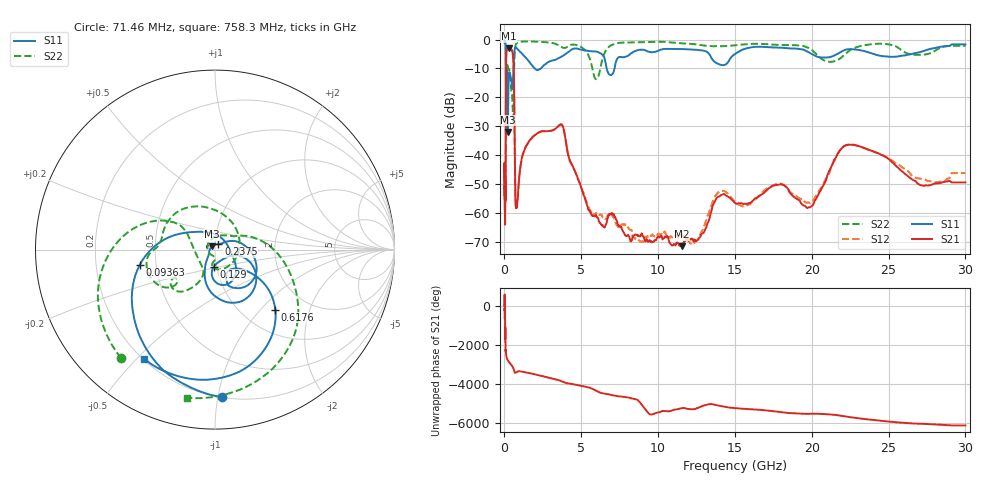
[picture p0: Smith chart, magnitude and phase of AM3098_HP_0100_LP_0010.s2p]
! Date/Time: Thu, Feb 28, 2019 8:35 AM
! Network Analyzer: Agilent Technologies E8364B Rev: A.07.50.67
! Sweep from 0.010 to 30.000 GHz, 1601 Points, Sweep Type: LOG
! Power Supply: 5.022 V, 0.002 A
# Hz S DB R 50
!freq MagS11 AngS11 MagS21 AngS21 MagS12 AngS12 MagS22 AngS22
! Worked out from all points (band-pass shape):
!   1601 points, 10 MHz to 30 GHz, reference 50 ohm
!   highest |S21| = -3.03 dB at 269.1 MHz (marker M1); lowest = -71.5 dB at 11.54 GHz (marker M2)
!   |S21| within 3 dB of the highest: 111.2 MHz to 562.7 MHz (451.5 MHz wide, 134 % of centre)
!   lowest |S11| = -32.0 dB at 229.3 MHz (marker M3), VSWR 1.05, Z = 48.3 + j1.78 ohm
!   |S11| at or under -10 dB: 176.3 MHz to 588 MHz (411.7 MHz wide, 108 % of centre); 1.966 GHz to 2.381 GHz (415.1 MHz wide, 19.1 % of centre); 6.65 GHz to 7.164 GHz (513.4 MHz wide, 7.43 % of centre)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
!   |S22| runs from -28.9 to -0.5 dB; largest |S21 - S12| = 0.012
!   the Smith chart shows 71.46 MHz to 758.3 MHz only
!   S11 on the Smith chart (normalised r, x): 71.46 MHz: 0.20, -1.03; 93.63 MHz: 0.40, -0.09; 129 MHz: 0.97, -0.19; 237.5 MHz: 1.04, +0.06; 617.6 MHz: 1.40, -1.21; 758.3 MHz: 0.21, -0.52
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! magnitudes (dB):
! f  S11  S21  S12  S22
! 10 MHz  -0.3  -42.9  -43.7  -0.5
! 38.04 MHz  -0.5  -60.1  -59.7  -0.8
! 71.46 MHz  -1.7  -54.4  -55.5  -1.9
! 93.63 MHz  -7.4  -21.8  -21.8  -8.7
! 129 MHz  -20.4  -4.3  -4.3  -10.8
! 144.7 MHz  -15.8  -3.7  -3.7  -10.8
! 186.8 MHz  -11.2  -3.5  -3.5  -8.2
! 229.3 MHz  -32.0  -3.1  -3.1  -9.9
! 237.5 MHz  -28.9  -3.1  -3.1  -10.0
! 269.1 MHz  -14.9  -3.0  -3.0  -10.4
! 550.5 MHz  -15.0  -5.4  -5.4  -25.1
! 617.6 MHz  -6.5  -13.4  -13.3  -13.2
! 758.3 MHz  -2.8  -58.2  -57.7  -1.5
! 2.084 GHz  -10.5  -32.7  -32.6  -0.7
! 3.723 GHz  -5.9  -29.5  -29.4  -2.6
! 5.989 GHz  -4.2  -61.1  -60.0  -13.7
! 7.926 GHz  -5.9  -68.1  -64.6  -1.0
! 11.54 GHz  -3.3  -71.5  -67.3  -1.3
! 14.16 GHz  -8.9  -53.7  -52.4  -2.3
! 19.8 GHz  -4.4  -58.0  -56.4  -3.0
! 22.56 GHz  -3.3  -36.4  -36.3  -3.5
! 30 GHz  -1.7  -49.4  -46.2  -2.2
